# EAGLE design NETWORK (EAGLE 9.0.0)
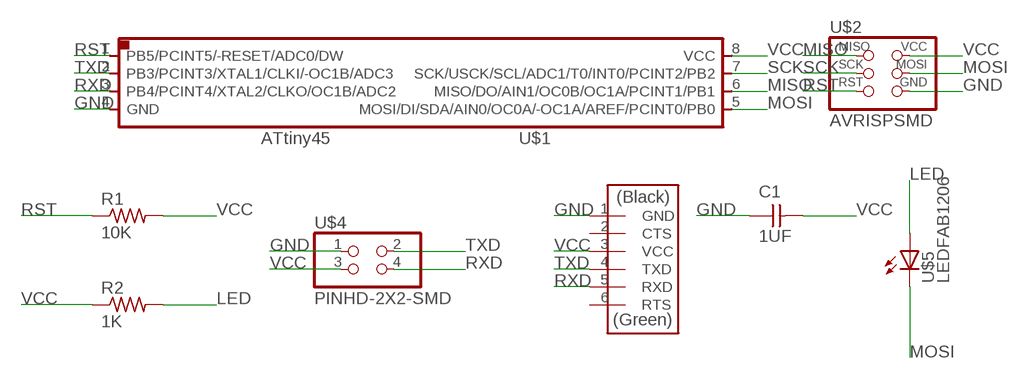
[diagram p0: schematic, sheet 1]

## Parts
C1  1UF  CAP-UNPOLARIZEDFAB  [C1206FAB]
R1  10K  RES-US1206FAB  [R1206FAB]
R2  1K  RES-US1206FAB  [R1206FAB]
U$1  ATTINY45SI  [SOIC8]
U$2  AVRISPSMD  [2X03SMD]
U$3  FTDI-SMD-HEADER  [1X06SMD]
U$4  PINHD-2X2-SMD  [2X02SMD]
U$5  LEDFAB1206  [LED1206FAB]

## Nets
GND: C1.1 U$1.4(GND) U$2.6(GND) U$3.1(GND) U$4.1
LED: R2.2 U$5.1(A)
MISO: U$1.6(MISO/DO/AIN1/OC0B/OC1A/PCINT1/PB1) U$2.1(MISO)
MOSI: U$1.5(MOSI/DI/SDA/AIN0/OC0A/-OC1A/AREF/PCINT0/PB0) U$2.4(MOSI) U$5.2(C)
RST: R1.1 U$1.1(PB5/PCINT5/-RESET/ADC0/DW) U$2.5(RST)
RXD: U$1.3(PB4/PCINT4/XTAL2/CLKO/OC1B/ADC2) U$3.5(RXD) U$4.4
SCK: U$1.7(SCK/USCK/SCL/ADC1/T0/INT0/PCINT2/PB2) U$2.3(SCK)
TXD: U$1.2(PB3/PCINT3/XTAL1/CLKI/-OC1B/ADC3) U$3.4(TXD) U$4.2
VCC: C1.2 R1.2 R2.1 U$1.8(VCC) U$2.2(VCC) U$3.3(VCC) U$4.3
Unconnected: U$3.2(CTS) U$3.6(RTS)

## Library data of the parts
C1 = fab:CAP-UNPOLARIZED
R1 R2 = fab:RES-US: Resistor (US Symbol)
U$1 = fab:ATTINY45
U$2 = fab:AVRISP
U$3 = fab:FTDI-SMD-HEADER
U$4 = fab:PINHD-2X2-SMD
U$5 = fab:LED: LED

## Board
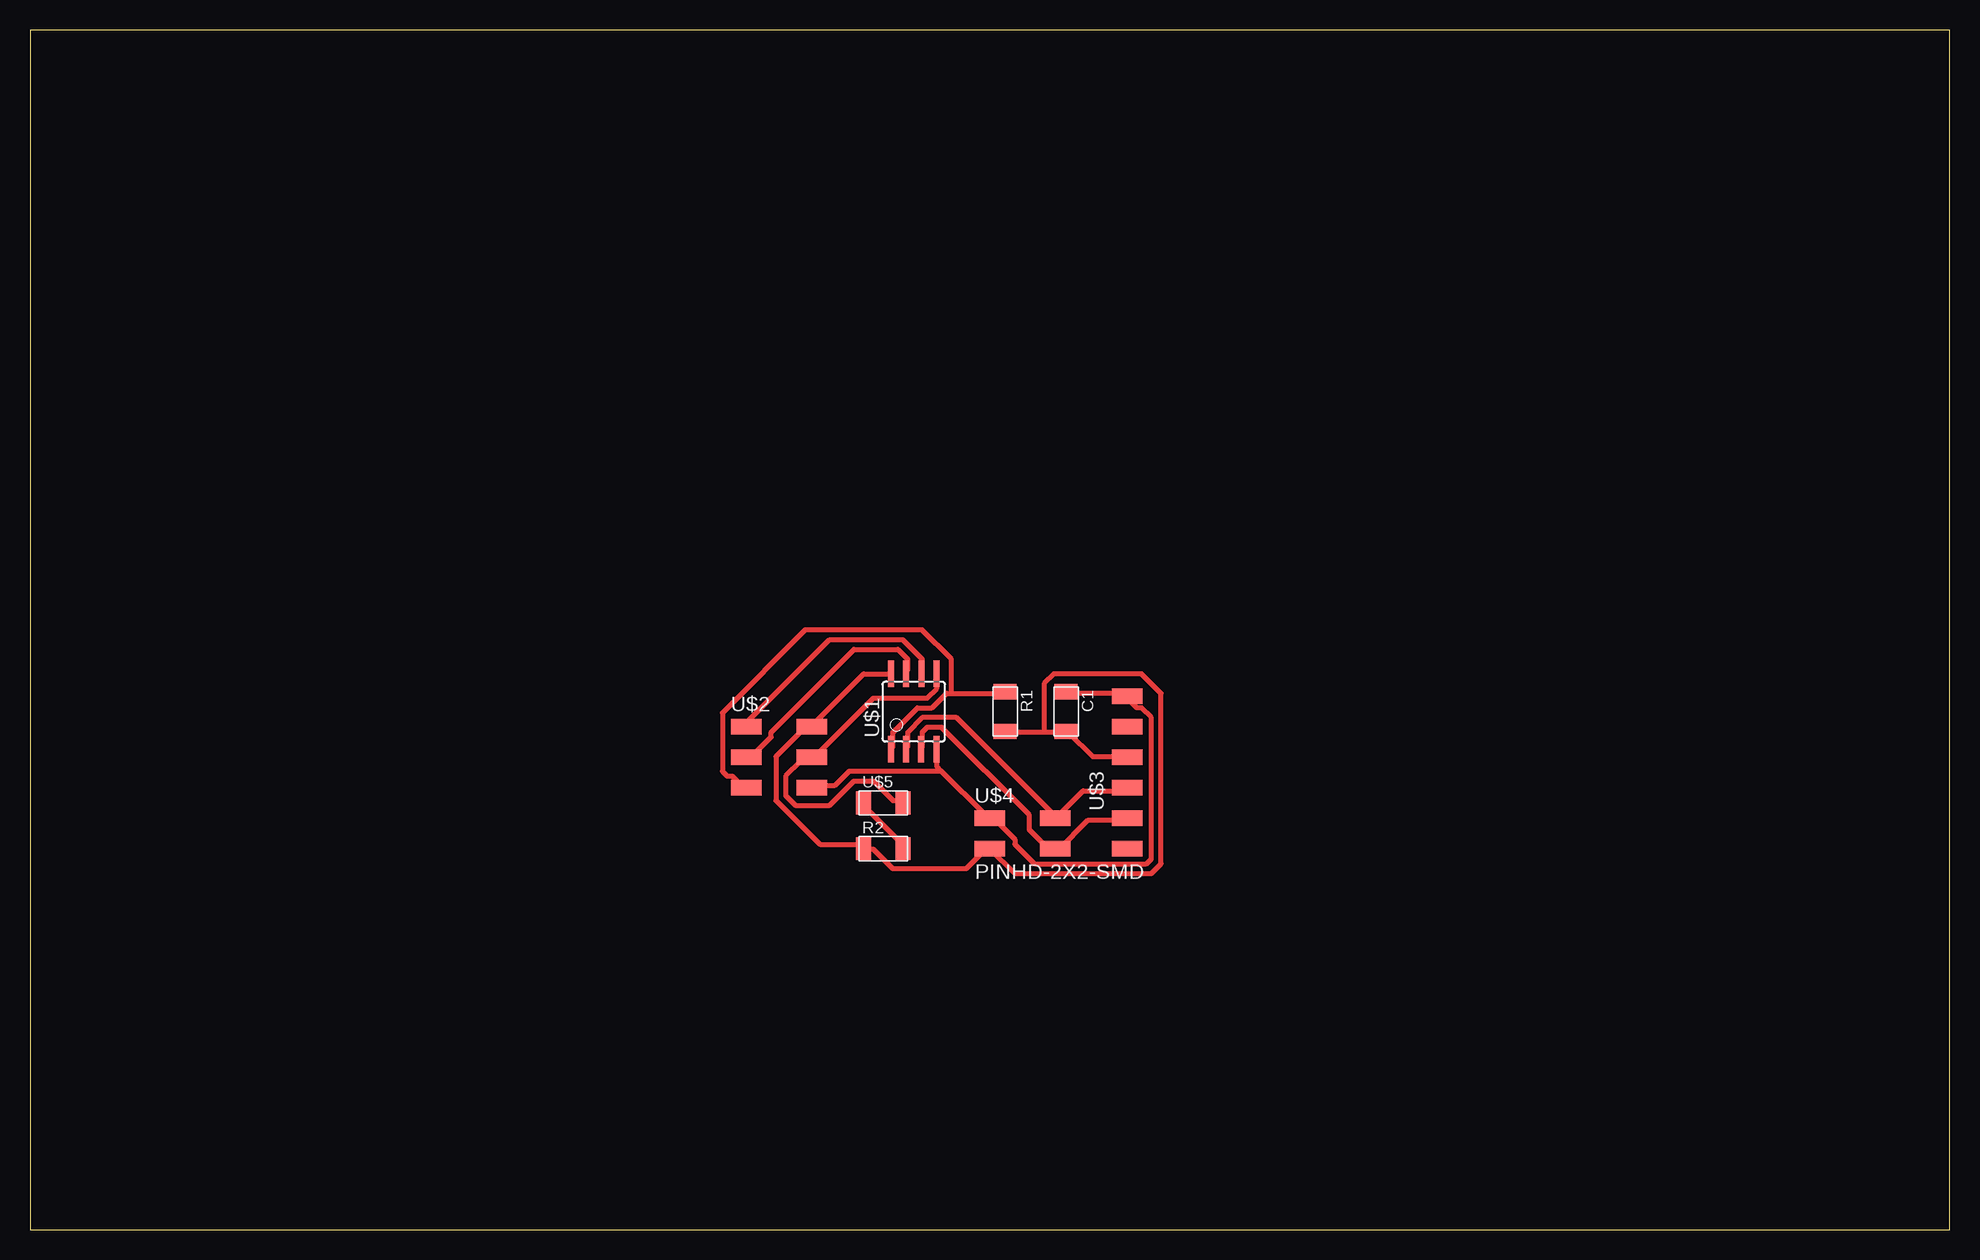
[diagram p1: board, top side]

Size 160 x 100 mm. Coordinates in mm from the lower left corner, seen from the top.
Outline: 0,0 160,0 160,100 0,100 0,0
Copper layers (1*16): Top 0.035mm / dielectric 1.5mm / Bottom 0.035mm
Design rules "default *": minimum track width 16mil, minimum drill 0.35mm, track to track 16mil, track to pad 16mil, pad to pad 16mil, via to via 16mil, smd to smd 16mil, copper to edge 40mil, drill to drill 6mil, minimum pad ring 10mil, minimum via ring 8mil, stop-mask expansion 4mil, vias tented up to drill 0mil, thermal gap 10mil

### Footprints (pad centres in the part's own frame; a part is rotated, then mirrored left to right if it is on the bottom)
C1206FAB = smd 1.27 x 1.905: 1 -1.651,0; 2 1.651,0
R1206FAB = smd 1.27 x 1.905: 1 -1.651,0; 2 1.651,0
SOIC8 = smd 0.5 x 2.2: 1 -1.905,-3.154; 2 -0.645,-3.154; 3 0.625,-3.154; 4 1.895,-3.154; 5 1.905,3.154; 6 0.635,3.154; 7 -0.635,3.154; 8 -1.905,3.154
2X03SMD = smd 2.54 x 1.27: 1 -2.54,2.54; 2 2.92,2.54; 3 -2.54,0; 4 2.92,0; 5 -2.54,-2.54; 6 2.92,-2.54
1X06SMD = smd 2.54 x 1.27: 1 0,6.35; 2 0,3.81; 3 0,1.27; 4 0,-1.27; 5 0,-3.81; 6 0,-6.35
2X02SMD = smd 2.54 x 1.27: 1 -2.54,1.27; 2 2.92,1.27; 3 -2.54,-1.27; 4 2.92,-1.27
LED1206FAB = smd 1.27 x 1.905: 1 -1.651,0; 2 1.651,0

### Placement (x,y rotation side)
C1  86.36,43.18 270 top
R1  81.28,43.18 270 top
R2  71.12,31.75 0 top
U$1  73.66,43.18 0 top
U$2  62.23,39.37 0 top
U$3  91.44,38.1 0 top
U$4  82.55,33.02 0 top
U$5  71.12,35.56 0 top

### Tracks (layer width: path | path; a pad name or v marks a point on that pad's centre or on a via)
GND
  Top 0.406: C1.1 86.56,44.7 91.44,44.7 U$3.1 91.44,44.3 92.25,43.48 92.66,43.48 93.47,42.67 93.47,30.89 93.07,30.48 83.72,30.48 82.09,32.11 82.09,32.51 80.06,34.54 U$4.1 79.65,34.54 76,38.2 | 76,38.2 75.59,38.61 75.59,39.83 U$1.4 | 76,38.2 68.28,38.2 67.06,36.98 65.43,36.98 U$2.6
LED
  Top 0.406: U$5.1 69.49,35.36 72.75,32.11 R2.2
MISO
  Top 0.406: U$1.6 74.37,46.74 74.37,47.55 72.75,49.17 66.65,49.17 59.74,42.27 U$2.1
MOSI
  Top 0.406: U$5.2 72.75,35.76 71.93,35.76 70.31,37.39 68.68,37.39 66.65,35.36 63.8,35.36 62.99,36.17 62.99,37.8 64.21,39.01 65.02,39.01 U$2.4 65.43,39.42 70.31,44.3 74.78,44.3 75.59,45.11 75.59,46.33 U$1.5
RST
  Top 0.406: 76.81,44.7 76.4,44.7 75.18,43.48 73.97,43.48 71.93,41.45 71.93,40.23 U$1.1 | 76.81,44.7 81.28,44.7 R1.1 | 76.81,44.7 76.81,47.55 74.37,49.99 64.62,49.99 57.71,43.08 57.71,38.2 58.12,37.8 58.52,37.8 59.33,36.98 U$2.5
RXD
  Top 0.406: U$1.3 74.37,40.23 74.37,41.45 74.78,41.86 76,41.86 83.31,34.54 83.31,33.33 84.53,32.11 85.34,32.11 U$4.4 85.75,31.7 88.19,34.14 91.44,34.14 U$3.5
SCK
  Top 0.406: U$1.7 73.15,46.74 73.15,47.55 72.34,48.36 68.68,48.36 61.77,41.45 61.77,41.05 59.74,39.01 U$2.3
TXD
  Top 0.406: U$1.2 73.15,40.23 73.15,41.45 74.37,42.67 77.22,42.67 85.34,34.54 U$4.2 85.75,34.54 87.78,36.58 91.44,36.58 U$3.4
VCC
  Top 0.406: 84.53,41.45 86.16,41.45 C1.2 86.56,41.45 88.59,39.42 91.44,39.42 U$3.3 | 84.53,41.45 81.28,41.45 R1.2 | U$1.8 71.53,46.33 69.49,46.33 65.43,42.27 U$2.2 65.02,42.27 62.18,39.42 62.18,35.76 65.84,32.11 69.09,32.11 R2.1 69.49,31.7 70.31,31.7 71.93,30.07 78.03,30.07 79.65,31.7 U$4.3 82.09,29.67 93.47,29.67 94.28,30.48 94.28,44.7 92.66,46.33 85.34,46.33 84.53,45.52 84.53,41.45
